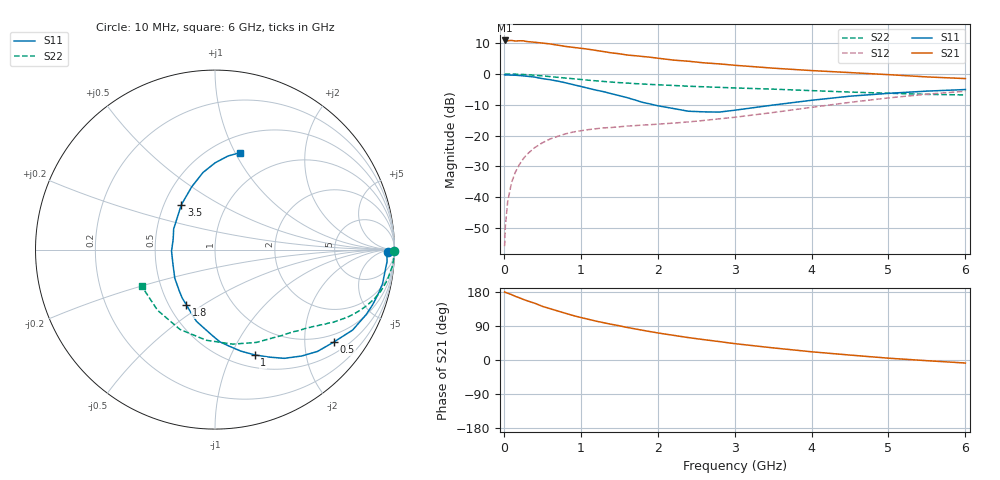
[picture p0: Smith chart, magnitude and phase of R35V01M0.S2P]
! SIEMENS Small Signal Semiconductors
! BFR181
! Si NPN RF Bipolar Junction Transistor in SOT23
! VCE = 5 V  IC = 1 mA
! Common Emitter S-Parameters:  May  1996
# GHz  S  MA  R  50
!  f  S11  S21  S12  S22
! GHz  MAG  ANG  MAG  ANG  MAG  ANG  MAG  ANG
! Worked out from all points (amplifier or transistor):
!   36 points, 10 MHz to 6 GHz, reference 50 ohm
!   highest |S21| = 10.9 dB at 10 MHz (marker M1)
!   |S21| within 3 dB of that: start of sweep to 1.137 GHz
!   unconditionally stable (mu >= 1): 2.04 GHz to 3.686 GHz
!   at 250 MHz: K = 0.16, MSG = 19.2 dB, |S12| = -27.6 dB
!   at 1.4 GHz: K = 0.77, MSG = 12.1 dB, |S12| = -17.4 dB
!   at 6 GHz: K = 0.87, MSG = 2.1 dB, |S12| = -5.6 dB
!   lowest NFmin = 1.30 dB at 450 MHz
!   S11 on the Smith chart (normalised r, x): 10 MHz: 45, -19; 500 MHz: 0.78, -2.72; 1 GHz: 0.64, -1.23; 1.8 GHz: 0.61, -0.43; 3.5 GHz: 0.61, +0.34; 6 GHz: 0.67, +1.05
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0.01  0.9631 -0.9  3.492 179.4  0.0016 93.9  0.9978 -0.3
0.02  0.9579 -1.6  3.412 178.4  0.0034 87.3  0.9907 -0.7
0.05  0.9611 -3.9  3.453 176.3  0.0085 88.9  0.9979 -1.8
0.1  0.9544 -7.8  3.492 172.6  0.0172 85.9  0.9958 -3.6
0.15  0.9527 -11.5  3.416 167.9  0.0255 81.8  0.9914 -5.6
0.25  0.9301 -19.4  3.449 160.2  0.0416 77.2  0.9788 -9.1
0.5  0.8393 -37.8  3.172 141.7  0.0761 66.3  0.9296 -17.1
0.6  0.805 -44.8  3.066 135.5  0.0877 62.3  0.9051 -19.8
0.7  0.7649 -50.8  2.933 129.4  0.0971 59.1  0.881 -22.3
0.9  0.6711 -63.2  2.699 117.4  0.114 53.5  0.8355 -26.4
1  0.6264 -69.4  2.608 112.2  0.1195 51.2  0.812 -28.3
1.1  0.5838 -75.7  2.513 107.4  0.1247 49.3  0.7905 -30.0
1.2  0.5451 -81.4  2.405 102.5  0.129 47.7  0.7719 -31.7
1.4  0.4767 -92.1  2.195 94.1  0.1351 45.4  0.7368 -34.5
1.8  0.3466 -117.4  1.921 78.6  0.1479 44.3  0.6866 -39.0
2.2  0.2751 -144.5  1.679 65.3  0.1589 45.6  0.6496 -44.0
2.4  0.2478 -161.1  1.606 59.1  0.1663 47.1  0.6313 -46.5
2.8  0.2401 166.0  1.455 48.6  0.1865 49.5  0.6056 -52.3
3.5  0.3124 126.9  1.24 32.0  0.2363 51.7  0.5662 -66.0
4.5  0.4351 98.8  1.051 13.0  0.3456 47.5  0.5074 -95.5
5.5  0.5259 82.2  0.894 -1.8  0.4688 35.3  0.4656 -133.5
6  0.5576 75.6  0.84 -8.0  0.5238 27.4  0.4564 -153.6
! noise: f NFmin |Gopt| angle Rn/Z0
0.45  1.3  0.7  18  0.5
0.9  1.4  0.6  39  0.52
1.8  1.85  0.4  81  0.47
